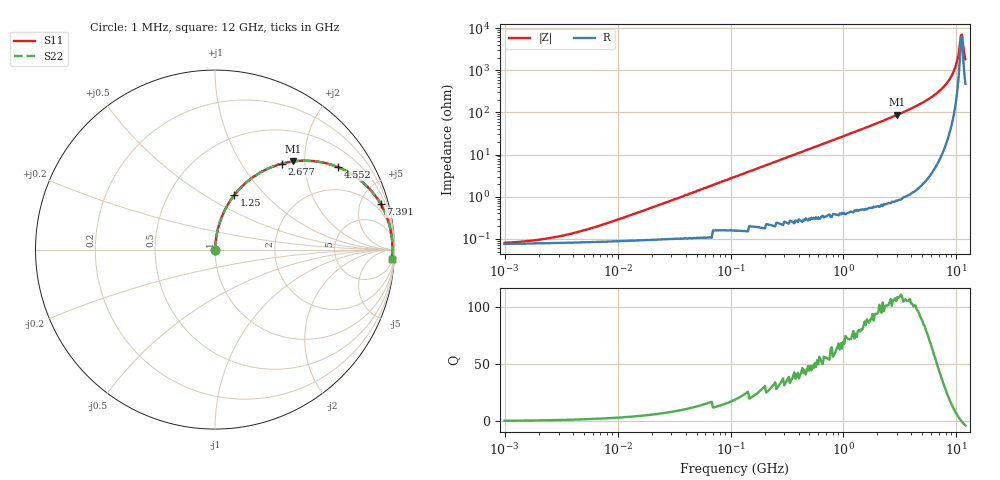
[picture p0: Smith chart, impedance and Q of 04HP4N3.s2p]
# MHz S MA R 50
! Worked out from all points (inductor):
!   408 points, 1 MHz to 12 GHz, reference 50 ohm
!   read as one part in series: L = 4.3 nH near 9.823 MHz
!   highest Q = 108 at 3.005 GHz (marker M1), where L = 4.64 nH
!   self-resonance near 10.94 GHz
!   S11 on the Smith chart (normalised r, x): 1 MHz: 1.00, +0.00; 1.25 GHz: 1.01, +0.68; 2.677 GHz: 1.02, +1.54; 4.552 GHz: 1.03, +2.96; 7.391 GHz: 1.19, +7.19; 12 GHz: 10, -35
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1  0.0005786 27.8  0.999 -0.0  0.999 -0.0  0.0005786 27.8
2.142  0.0008075 45.7  0.999 -0.0  0.999 -0.0  0.0008075 45.7
4.803  0.001448 63.5  0.999 -0.1  0.999 -0.1  0.001448 63.5
23.071  0.006297 81.1  0.999 -0.4  0.999 -0.4  0.006297 81.1
110.816  0.03 85.3  0.998 -1.7  0.998 -1.7  0.03 85.3
532.275  0.142 80.6  0.987 -8.2  0.987 -8.2  0.142 80.6
1250.174  0.322 70.4  0.942 -18.8  0.942 -18.8  0.322 70.4
1808.554  0.447 62.8  0.89 -26.5  0.89 -26.5  0.447 62.8
2556.642  0.587 53.5  0.804 -35.9  0.804 -35.9  0.587 53.5
2677.41  0.606 52.1  0.789 -37.3  0.789 -37.3  0.606 52.1
3004.884  0.656 48.5  0.749 -41.0  0.749 -41.0  0.656 48.5
4552.331  0.825 33.9  0.557 -55.5  0.557 -55.5  0.825 33.9
6004.882  0.912 23.4  0.397 -65.7  0.397 -65.7  0.912 23.4
7391.073  0.957 15.4  0.266 -73.0  0.266 -73.0  0.957 15.4
8488.733  0.976 10.1  0.176 -77.2  0.176 -77.2  0.976 10.1
9309.645  0.984 6.6  0.116 -78.7  0.116 -78.7  0.984 6.6
9977.019  0.987 4.0  0.07 -77.5  0.07 -77.5  0.987 4.0
10692.23  0.988 1.4  0.026 -62.5  0.026 -62.5  0.988 1.4
10941.86  0.988 0.5  0.015 -34.7  0.015 -34.7  0.988 0.5
11197.31  0.987 -0.4  0.014 27.7  0.014 27.7  0.987 -0.4
11458.72  0.987 -1.3  0.025 58.0  0.025 58.0  0.987 -1.3
12000  0.985 -3.0  0.054 72.0  0.054 72.0  0.985 -3.0
